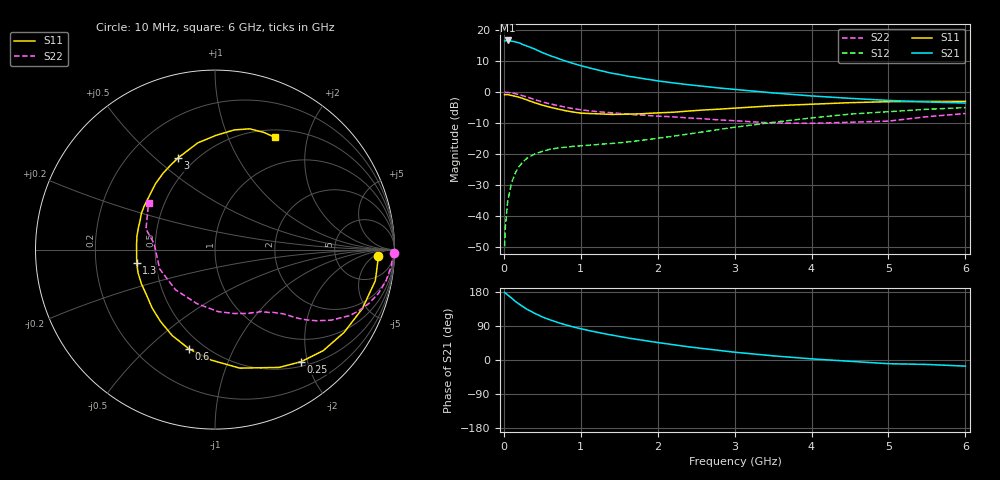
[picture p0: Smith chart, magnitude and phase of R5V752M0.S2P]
! SIEMENS Small Signal Semiconductors
! BFR183
! Si NPN RF Bipolar Junction Transistor in SOT23
! VCE = 0.75 V  IC = 2 mA
! Common Emitter S-Parameters:  May  1996
# GHz  S  MA  R  50
!  f  S11  S21  S12  S22
! GHz  MAG  ANG  MAG  ANG  MAG  ANG  MAG  ANG
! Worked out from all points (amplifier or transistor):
!   36 points, 10 MHz to 6 GHz, reference 50 ohm
!   highest |S21| = 16.6 dB at 50 MHz (marker M1)
!   |S21| within 3 dB of that: start of sweep to 421.9 MHz
!   unconditionally stable (mu >= 1): 1.342 GHz to 3.208 GHz
!   at 250 MHz: K = 0.24, MSG = 18.9 dB, |S12| = -22.5 dB
!   at 1.4 GHz: K = 1.03, MAG = 10.2 dB, |S12| = -16.6 dB
!   at 6 GHz: K = 0.97, MSG = 0.7 dB, |S12| = -5.0 dB
!   S11 on the Smith chart (normalised r, x): 10 MHz: 18, -8; 250 MHz: 0.58, -1.89; 600 MHz: 0.42, -0.68; 1.3 GHz: 0.39, -0.07; 3 GHz: 0.41, +0.60; 6 GHz: 0.60, +1.50
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0.01  0.9108 -2.2  6.652 178.7  0.0033 89.8  0.9951 -1.0
0.02  0.9092 -4.4  6.69 176.6  0.0068 86.7  0.9901 -2.0
0.05  0.91 -11.0  6.784 171.6  0.0174 83.2  0.9873 -5.2
0.1  0.8842 -21.9  6.622 163.6  0.0344 77.9  0.9688 -10.3
0.15  0.8543 -32.7  6.43 154.7  0.0501 71.4  0.9424 -15.1
0.2  0.825 -43.0  6.204 147.4  0.0639 66.5  0.9082 -19.3
0.25  0.7878 -52.4  5.814 140.6  0.0752 61.3  0.87 -23.1
0.3  0.7476 -61.4  5.509 134.0  0.0859 57.6  0.8357 -26.1
0.4  0.6746 -78.2  4.946 123.3  0.1006 50.5  0.7585 -31.2
0.5  0.6157 -92.1  4.325 113.7  0.111 45.6  0.6929 -34.9
0.6  0.5712 -104.8  3.869 106.0  0.1198 42.2  0.6474 -37.3
0.8  0.5016 -127.5  3.162 92.9  0.1296 38.0  0.5712 -40.9
0.9  0.4777 -137.3  2.899 87.4  0.1335 37.5  0.5408 -42.2
1.1  0.4522 -155.0  2.473 78.0  0.1392 37.0  0.5012 -45.0
1.3  0.4426 -170.3  2.153 69.7  0.146 37.3  0.4744 -47.4
1.6  0.4414 170.2  1.814 58.5  0.1568 39.7  0.4429 -51.7
2.2  0.4735 140.3  1.407 40.4  0.1947 44.5  0.3992 -63.1
3  0.5509 111.9  1.105 20.6  0.2716 44.2  0.3459 -87.1
3.5  0.6022 99.2  0.97 11.0  0.3262 40.0  0.3173 -108.6
4.5  0.6755 80.8  0.793 -3.4  0.4418 27.7  0.3266 -160.7
5.5  0.7073 67.4  0.693 -11.7  0.5283 14.2  0.401 163.5
6  0.7091 61.9  0.667 -16.2  0.5628 5.6  0.452 145.0
